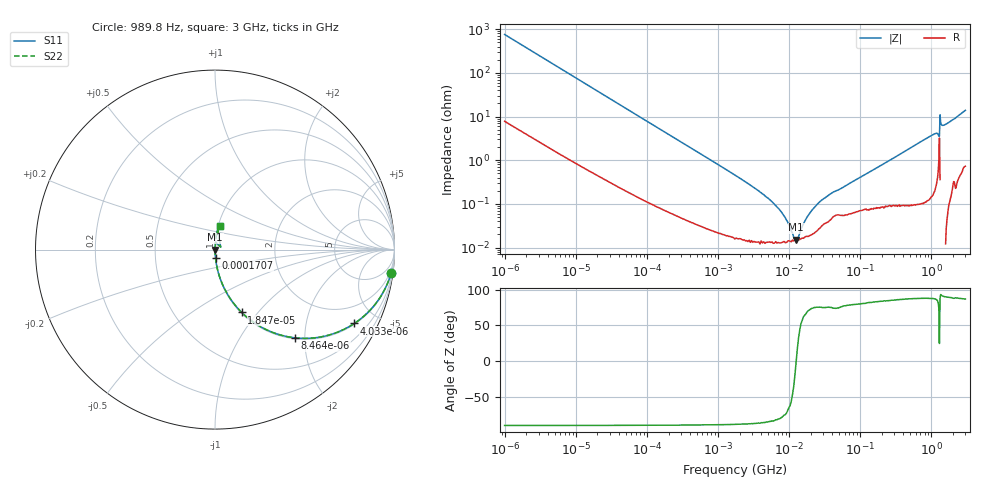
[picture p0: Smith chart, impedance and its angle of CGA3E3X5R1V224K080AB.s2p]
! S-Parameter Data Generated by TDK Corporation
! Copyright(C) 2020 TDK Corporation.
! All Rights Reserved.
! TDK P/N: CGA3E3X5R1V224K080AB (Multilayer Ceramic Chip Capacitor)
! Property: C=220nF
! Size(LxWxT): 1.6x0.8x0.8mm
! Model Type: s2p (Touchstone File Format Version 1.0)
! Frequency: DC=Yes Start=0.000989846MHz Stop=3000MHz 463points Log-sweep
! Model Generated on Aug. 18, 2020
! Port Assignments:
!  1 ---| |--- 2
! Applicable Conditions:
!  Temperature = 25 degC
!  DC Bias Voltage = 0 V
!  Small Signal Operation
! Terms and conditions regarding TDK Simulation Models
! (1)This simulation model is being provided solely for informational purposes. Please refer to the specifications of the products in terms of detailed characteristics of such products.
! (2)In no event shall TDK Corporation of any of its subsidiaries be liable for any loss or damage arising, directly or indirectly,
!  From any information contained in this simulation model, including, but not limited to loss or damages arising from any inaccuracies, omissions or errors in connection with such information.
! (3)Any and all copyrights on this simulation model are owned by TDK Corporation.
!  Duplication or redistribution of this simulation model without prior written permission from TDK Corporation is prohibited.
! (4)This simulation model is subject to any modification or change without any prior notice.
! (5)Neither TDK Corporation nor any of its subsidiaries shall make any warranty, express or implied,
!  Including but not limited to the correctness, implied warranties of merchantability and fitness for a particular purpose with respect to this simulation models.
! (6)The use of this simulation model shall be deemed to have consented to the terms and conditions hereof.
# Hz S MA R 50
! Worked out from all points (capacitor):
!   462 points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, 989.8 Hz to 3 GHz, reference 50 ohm
!   read as one part in series: C = 212 nF near 1.07 kHz
!   lowest |Z| = 15.1 mohm at 12.48 MHz (marker M1)
!   series resonance near 12.51 MHz, so ESL is about 760 pH
!   S11 on the Smith chart (normalised r, x): 989.8 Hz: 1, -15; 4.033 kHz: 1.04, -3.75; 8.464 kHz: 1.02, -1.80; 18.47 kHz: 1.01, -0.83; 170.7 kHz: 1.00, -0.09; 3 GHz: 1.01, +0.28
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989.846  0.9901 -7.5  0.1306 81.9  0.1306 81.9  0.9901 -7.5
2246.057  0.9557 -16.5  0.2847 72.9  0.2847 72.9  0.9557 -16.5
4032.751  0.8786 -27.9  0.4684 61.5  0.4684 61.5  0.8786 -27.9
8463.765  0.6644 -47.7  0.7401 41.6  0.7401 41.6  0.6644 -47.7
12024.64  0.5324 -57.2  0.8406 32.2  0.8406 32.2  0.5324 -57.2
18470.18  0.3808 -67.0  0.9203 22.4  0.9203 22.4  0.3808 -67.0
40306.84  0.1873 -78.5  0.98 10.8  0.98 10.8  0.1873 -78.5
146075.1  0.0534 -86.1  0.9978 3.1  0.9978 3.1  0.0534 -86.1
170748.8  0.04578 -86.5  0.9982 2.6  0.9982 2.6  0.04578 -86.5
1774518  0.004427 -87.6  0.9998 0.3  0.9998 0.3  0.004427 -87.6
6184898  0.0009856 -82.6  0.9999 0.1  0.9999 0.1  0.0009856 -82.6
8450755  0.0005289 -74.8  0.9999 0.0  0.9999 0.0  0.0005289 -74.8
1.154672e7  0.0001723 -34.9  0.9999 0.0  0.9999 0.0  0.0001723 -34.9
1.248387e7  0.0001507 -0.9  0.9998 0.0  0.9998 0.0  0.0001507 -0.9
2.073191e7  0.0007116 73.8  0.9998 -0.0  0.9998 -0.0  0.0007116 73.8
3.870484e7  0.001735 75.1  0.9996 -0.1  0.9996 -0.1  0.001735 75.1
2.507343e8  0.009674 84.1  0.9991 -0.6  0.9991 -0.6  0.009674 84.1
1.017911e9  0.03745 85.6  0.9978 -2.1  0.9978 -2.1  0.03745 85.6
1.243477e9  0.03912 79.5  0.9936 -2.2  0.9936 -2.2  0.03912 79.5
1.374365e9  0.06545 88.5  1 -3.7  1 -3.7  0.06545 88.5
1.581072e9  0.06621 86.1  0.9977 -3.8  0.9977 -3.8  0.06621 86.1
3e9  0.1366 79.1  0.9835 -7.8  0.9835 -7.8  0.1366 79.1
